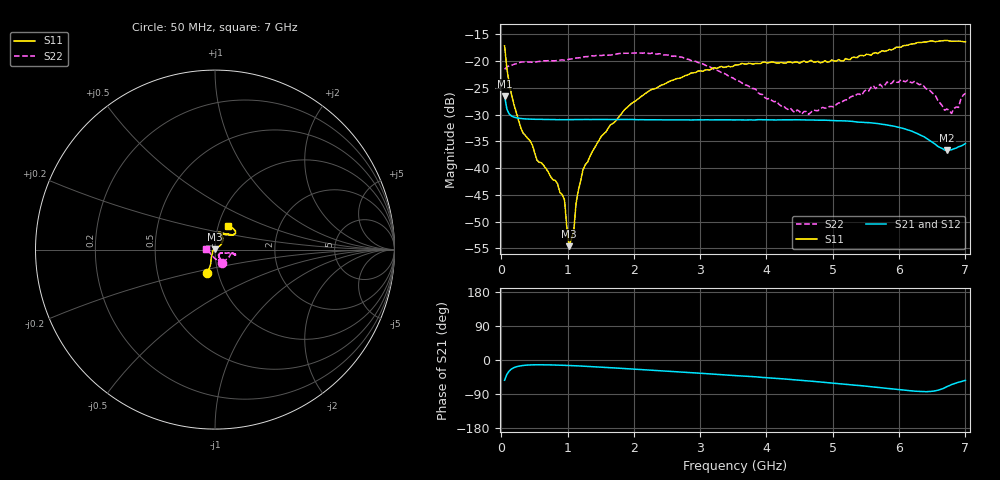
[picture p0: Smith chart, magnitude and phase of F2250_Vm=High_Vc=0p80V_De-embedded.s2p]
! Integrated Device Technology
! Corporate Headquarters
! 6024 Silver Creek Valley Road
! San Jose, CA 95138  USA
! Phone:  1-408-284-8200
! Toll Free:  1-800-223-1366
! Webpage:  http://www.idt.com/
! Timing and RF Division
! 515 Groton Road, Suite 102
! Westford, MA 01886-6024
! Device:  F2250
! Description: Voltage Variable RF Attenuator
! Frequency:  50.0 -  6000.00 MHz
! Package:  3x3 mm Thin QFN Plastic Package: 16 pin
! Ports:  2 RF, 3 DC
!  Pin  1  = GND
!  Pin  2  = NC
!  Pin  3  = RF1  = Port 1
!  Pin  4  = NC
!  Pin  5  = GND
!  Pin  6  = GND
!  Pin  7  = GND
!  Pin  8  = GND
!  Pin  9  = NC
!  Pin 10  = RF2  = Port 2
!  Pin 11  = NC
!  Pin 12  = GND
!  Pin 13  = GND
!  Pin 14  = VCNTRL
!  Pin 15  = VDD
!  Pin 16  = VMODE
! Vcntrl:  0.800 Volts
! Vmode:  +3.300 Volts
! Vdd:  +3.30  Volts
! Current:  1.303 mA
! Data:  The device was measured on a the F2250 evaluation board which has
!  individual transmission lines to the RF pins.  Data was collected
!  using a calibrated network analyzer.  The evaluation board was
!  de-embedded using a TRL calibration technique.
!  The reference plane is the edge of the package pin.
! Misc:  SN 10
!  Action Tracker AT0258
! Date Measured:  2014-11-26
! Date:  2015-10-15  MJV
! Note:
!  Integrated Device Technology supplies this data as a sample of measured
!  data at the package pin for this product.  Your particular data for this
!  product may vary.
!  Data was taken at 25 degrees C.
!  Integrated Device Technology reserves the right to change this data at anytime.
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# GHz S dB R 50
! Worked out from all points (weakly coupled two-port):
!   201 points, 50 MHz to 7 GHz, reference 50 ohm
!   highest |S21| = -26.55 dB at 50 MHz (marker M1); lowest = -36.7 dB at 6.722 GHz (marker M2)
!   lowest |S11| = -54.6 dB at 1.023 GHz (marker M3), VSWR 1.00, Z = 49.9 + j0.144 ohm
!   |S11| at or under -10 dB: start of sweep to end of sweep
!   |S22| runs from -30.0 to -18.4 dB; largest |S21 - S12| = 0.00012
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0.05  -17.14 -107.7  -26.55 -53.3  -26.54 -53.3  -21.52 -60.3
0.1195  -24.21 -110.8  -29.88 -29.0  -29.86 -28.9  -20.89 -18.2
0.29325  -32.43 -124.9  -30.72 -15.3  -30.71 -15.3  -20.17 -10.0
0.467  -35.64 -143.3  -30.85 -12.8  -30.85 -12.8  -20.21 -7.7
0.5365  -38.49 -151.2  -30.89 -12.6  -30.87 -12.6  -20.10 -8.5
0.8145  -42.29 171.1  -30.93 -13.3  -30.93 -13.3  -19.93 -10.8
0.9535  -45.95 173.6  -30.94 -14.1  -30.93 -14.1  -19.83 -12.3
1.023  -54.60 129.1  -30.93 -14.5  -30.94 -14.5  -19.63 -12.5
1.0925  -51.86 64.8  -30.93 -15.0  -30.92 -15.0  -19.55 -12.8
1.12725  -46.64 47.2  -30.92 -15.3  -30.91 -15.3  -19.42 -13.3
1.2315  -40.35 34.7  -30.91 -16.2  -30.92 -16.2  -19.22 -14.5
1.6485  -31.90 38.8  -30.92 -20.3  -30.94 -20.3  -18.86 -14.7
1.96125  -27.94 39.3  -30.90 -23.7  -30.92 -23.7  -18.49 -14.8
2.37825  -24.74 45.6  -30.95 -28.2  -30.96 -28.2  -18.61 -13.9
3.525  -20.72 71.2  -30.99 -41.0  -30.99 -41.1  -23.39 -17.2
4.4285  -20.18 74.3  -30.95 -52.4  -30.96 -52.4  -29.61 -41.5
4.7065  -20.14 71.7  -31.01 -56.3  -31.02 -56.3  -29.12 -49.7
5.85325  -17.83 40.2  -32.02 -75.5  -32.02 -75.5  -24.27 -62.8
6.33975  -16.51 40.5  -33.94 -83.1  -33.91 -83.3  -24.29 -76.4
6.722  -16.13 49.0  -36.66 -70.1  -36.65 -70.3  -28.95 -129.0
6.7915  -16.29 51.0  -36.57 -64.9  -36.58 -64.9  -29.78 -145.5
7  -16.39 62.1  -35.41 -53.8  -35.39 -53.9  -26.02 174.4
